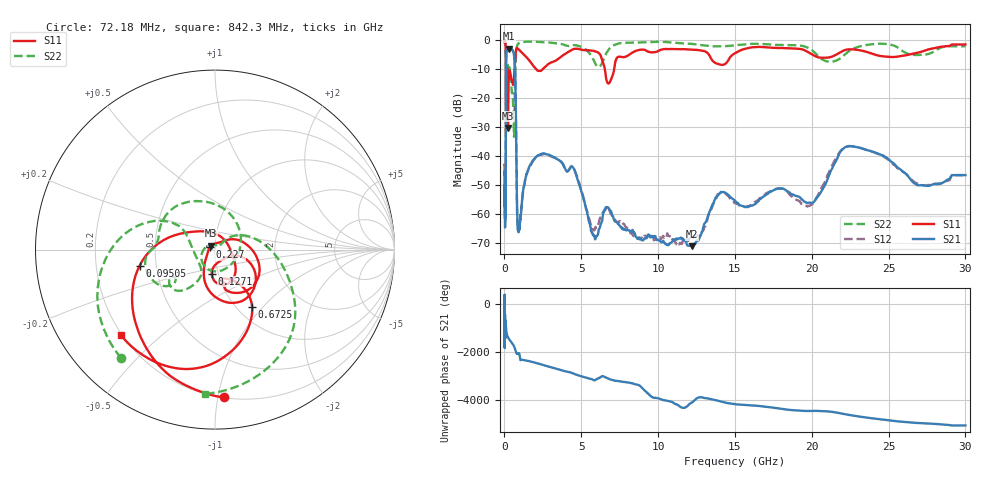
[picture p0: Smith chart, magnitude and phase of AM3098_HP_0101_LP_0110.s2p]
! Date/Time: Thu, Feb 28, 2019 8:36 AM
! Network Analyzer: Agilent Technologies E8364B Rev: A.07.50.67
! Sweep from 0.010 to 30.000 GHz, 1601 Points, Sweep Type: LOG
! Power Supply: 5.022 V, 0.002 A
# Hz S DB R 50
!freq MagS11 AngS11 MagS21 AngS21 MagS12 AngS12 MagS22 AngS22
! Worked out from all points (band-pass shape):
!   1601 points, 10 MHz to 30 GHz, reference 50 ohm
!   highest |S21| = -3.10 dB at 266.5 MHz (marker M1); lowest = -71.0 dB at 12.19 GHz (marker M2)
!   |S21| within 3 dB of the highest: 113.3 MHz to 641 MHz (527.6 MHz wide, 140 % of centre)
!   lowest |S11| = -30.4 dB at 229.3 MHz (marker M3), VSWR 1.06, Z = 47.9 + j2.11 ohm
!   |S11| at or under -10 dB: 176.7 MHz to 655.7 MHz (479 MHz wide, 115 % of centre); 2.03 GHz to 2.522 GHz (492.3 MHz wide, 21.6 % of centre); 6.526 GHz to 7.146 GHz (619.4 MHz wide, 9.06 % of centre)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
!   |S22| runs from -33.4 to -0.5 dB; largest |S21 - S12| = 0.011
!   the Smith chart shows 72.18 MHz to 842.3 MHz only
!   S11 on the Smith chart (normalised r, x): 72.18 MHz: 0.20, -1.04; 95.05 MHz: 0.40, -0.09; 127.1 MHz: 0.93, -0.25; 227 MHz: 0.94, +0.03; 672.5 MHz: 1.17, -0.88; 842.3 MHz: 0.20, -0.37
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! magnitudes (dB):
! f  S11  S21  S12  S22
! 10 MHz  -0.3  -46.3  -43.5  -0.5
! 38.04 MHz  -0.5  -61.5  -59.0  -0.9
! 72.18 MHz  -1.7  -53.8  -53.1  -2.0
! 81.39 MHz  -2.5  -52.0  -50.3  -2.7
! 95.05 MHz  -7.3  -22.5  -22.5  -8.6
! 127.1 MHz  -17.4  -4.7  -4.7  -10.3
! 144.7 MHz  -16.6  -3.8  -3.8  -10.9
! 184.9 MHz  -10.9  -3.6  -3.6  -8.0
! 227 MHz  -30.0  -3.2  -3.2  -9.5
! 229.3 MHz  -30.4  -3.2  -3.2  -9.5
! 266.5 MHz  -15.0  -3.1  -3.1  -9.8
! 550.5 MHz  -15.5  -3.9  -3.9  -20.4
! 620.7 MHz  -13.1  -5.3  -5.2  -33.4
! 672.5 MHz  -8.4  -8.3  -8.3  -19.3
! 842.3 MHz  -3.0  -61.6  -63.1  -1.9
! 2.084 GHz  -10.4  -40.2  -40.2  -0.8
! 7.926 GHz  -5.8  -65.6  -64.8  -1.1
! 12.19 GHz  -3.5  -71.0  -68.5  -1.5
! 14.09 GHz  -8.7  -52.3  -52.6  -2.3
! 19.8 GHz  -4.5  -56.1  -57.2  -2.9
! 22.67 GHz  -3.4  -36.7  -36.7  -3.2
! 30 GHz  -1.7  -46.6  -46.6  -2.3
